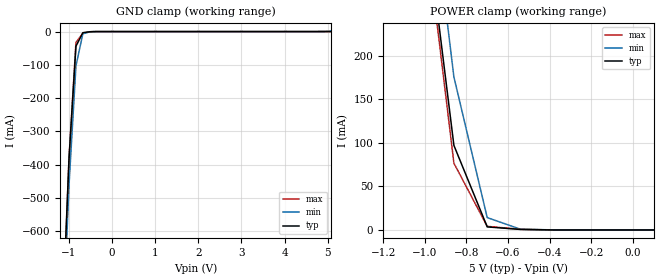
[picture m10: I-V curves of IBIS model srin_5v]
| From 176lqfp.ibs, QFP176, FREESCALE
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[Model] srin_5v
|   Model srin_5v
Model_type Input
Polarity   Non-Inverting
Enable   Active-High
Vinl =   1.7500V
Vinh =   3.2500V
C_comp   4.6867pF   4.5022pF   4.9393pF
[Temperature Range]   25.0000   0.1500k   -40.0000
[Voltage Range]   5.0000V   4.5000V   5.5000V
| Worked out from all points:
|   GND clamp passes 1 mA (typ) near -0.55 V on its own axis
|   POWER clamp passes 1 mA (typ) near -0.56 V on its own axis
[GND_clamp]
|Voltage   I(typ)   I(min)   I(max)
-5V       -15.48A    -15.42A    -15.57A
-1.16V    -883.1mA   -945.9mA   -900.9mA
-1V       -378.6mA   -458.6mA   -378.6mA
-840mV    -44.11mA   -102.9mA   -32.54mA
-680mV    -3.439mA   -6.731mA   -5.118mA
-520mV    -530.1uA   -781.9uA   -565.9uA
-360mV    -4.994uA   -45.89uA   -1.591uA
5.08V     230.9pA    1.498mA    9.384pA
[POWER_clamp]
|Voltage   I(typ)   I(min)   I(max)
-5V       11.12A     11.24A     11.12A
-1.02V    405.3mA    491.3mA    392.9mA
-860mV    97.05mA    175.5mA    76.65mA
-700mV    3.541mA    14.18mA    4.132mA
-540mV    594.7uA    858.4uA    774uA
100mV     54.85pA    7.446nA    9.775pA
